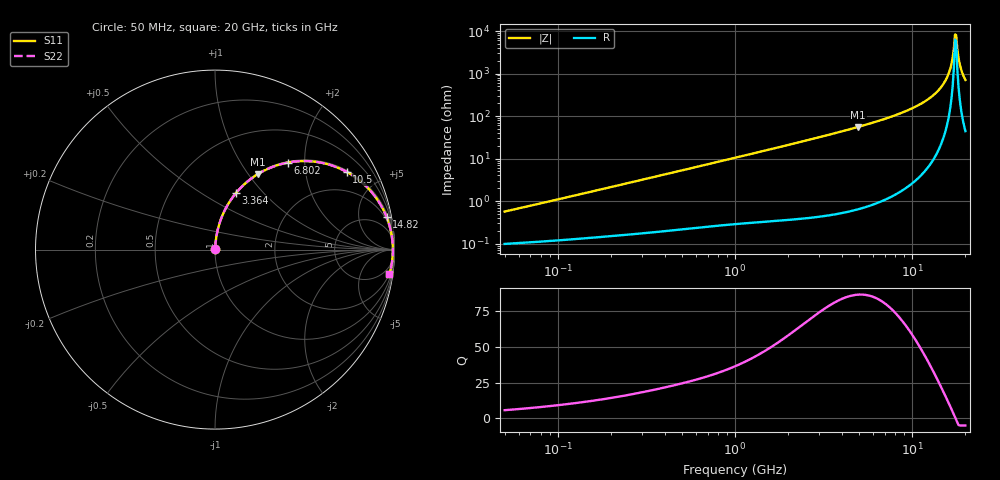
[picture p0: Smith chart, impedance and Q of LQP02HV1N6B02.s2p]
!Murata Part Number: LQP02HV1N6B02
!These Parameters are Measured in Series Mode Connection
!  o--[Z]--o
!Port1  Port2
!  o-------o
!Freq. Start=50[MHz] Stop=20[GHz], 401[Steps]
# Hz S RI R 50
!Freq.(Hz) S11(Real) S11(Imag) S21(Real) S21(Imag) S12(Real) S12(Imag) S22(Real) S22(Imag)
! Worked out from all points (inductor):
!   401 points, 50 MHz to 20 GHz, reference 50 ohm
!   read as one part in series: L = 1.76 nH near 51.52 MHz
!   highest Q = 86.5 at 4.967 GHz (marker M1), where L = 1.78 nH
!   self-resonance near 17.48 GHz
!   S11 on the Smith chart (normalised r, x): 50 MHz: 1.00, +0.01; 3.364 GHz: 1.01, +0.72; 6.802 GHz: 1.02, +1.65; 10.5 GHz: 1.06, +3.36; 14.82 GHz: 2, +10; 20 GHz: 2, -14
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5e7  0.00101 0.00557  0.999 -0.00557  0.999 -0.00557  0.00101 0.00557
1.364002e8  0.00153 0.0147  0.9985 -0.0147  0.9985 -0.0147  0.00153 0.0147
3.721004e8  0.00343 0.0391  0.9966 -0.0391  0.9966 -0.0391  0.00343 0.0391
1e9  0.0135 0.1025  0.9865 -0.1025  0.9865 -0.1025  0.0135 0.1025
2.728004e9  0.0799 0.2641  0.9201 -0.2641  0.9201 -0.2641  0.0799 0.2641
3.364474e9  0.1177 0.316  0.8823 -0.316  0.8823 -0.316  0.1177 0.316
4.966507e9  0.2385 0.4204  0.7615 -0.4204  0.7615 -0.4204  0.2385 0.4204
6.802353e9  0.4051 0.4848  0.5949 -0.4848  0.5949 -0.4848  0.4051 0.4848
7.442007e9  0.4657 0.4924  0.5343 -0.4924  0.5343 -0.4924  0.4657 0.4924
1.050288e10  0.7343 0.4326  0.2657 -0.4326  0.2657 -0.4326  0.7343 0.4326
1.276073e10  0.8778 0.314  0.1222 -0.314  0.1222 -0.314  0.8778 0.314
1.482269e10  0.9565 0.1807  0.0435 -0.1807  0.0435 -0.1807  0.9565 0.1807
1.550395e10  0.9719 0.1353  0.0281 -0.1353  0.0281 -0.1353  0.9719 0.1353
1.621653e10  0.9829 0.0883  0.0171 -0.0883  0.0171 -0.0883  0.9829 0.0883
1.670968e10  0.9877 0.0563  0.0123 -0.0563  0.0123 -0.0563  0.9877 0.0563
1.721783e10  0.9904 0.024  0.00963 -0.024  0.00963 -0.024  0.9904 0.024
1.747767e10  0.9909 0.00776  0.00908 -0.00776  0.00908 -0.00776  0.9909 0.00776
1.774144e10  0.9909 -0.00848  0.00906 0.00848  0.00906 0.00848  0.9909 -0.00848
1.800918e10  0.9904 -0.0247  0.00958 0.0247  0.00958 0.0247  0.9904 -0.0247
1.88369e10  0.9857 -0.0731  0.0143 0.0731  0.0143 0.0731  0.9857 -0.0731
1.940974e10  0.9799 -0.1049  0.0201 0.1049  0.0201 0.1049  0.9799 -0.1049
2e10  0.9722 -0.1361  0.0278 0.1361  0.0278 0.1361  0.9722 -0.1361
